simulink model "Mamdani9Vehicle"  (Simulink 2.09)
settings: Solver=ode45  StartTime=0.0  StopTime=50  MaxStep=10  RelTol=1e-3  AbsTol=1e-3
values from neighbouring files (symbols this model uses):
  vd = 45    [VdataM.m]
undefined symbols (not defined in the file or in its folder): sfunyst
libraries: fuzzy x4

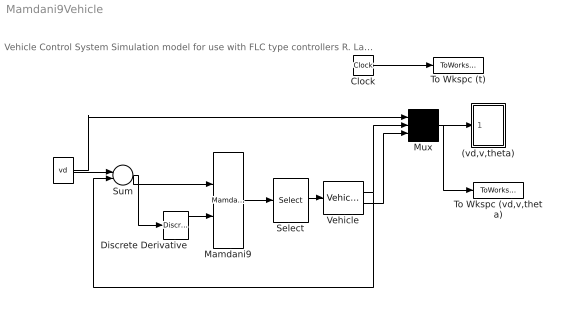
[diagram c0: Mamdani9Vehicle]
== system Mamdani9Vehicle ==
  note: Vehicle Control System Simulation model for use with FLC type controllers R. Langari 3/1/97
  " " : Constant  Value=vd
  (vd,v,theta) : Subsystem  mask(Storage scope.){}
      mask help: Storage scope using MATLAB graph window. Enter plotting ranges and line type.
      mask init:
      | npts = @4; color = @5; ax = [0, @1, @2, @3]; dt=-1;
  Clock : Clock
  Discrete Derivative : fuzzy/Discrete Derivative
  Mamdani9 : fuzzy/Mamdani9
  Mux : Mux  Inputs=3
  Select : fuzzy/Select
  Sum : Sum  Inputs=+-
  To Wkspc (vd,v,theta) : ToWorkspace  VariableName=yout  SampleTime=0
  To Wkspc (t) : ToWorkspace  VariableName=t  SampleTime=0
  Vehicle : fuzzy/Vehicle
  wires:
  Select/1 -> Vehicle/1
  Mux/1 -> (vd,v,theta)/1(x), To Wkspc (vd,v,theta)/1
  Vehicle/1 -> Sum/2, Mux/2
  Vehicle/2 -> Mux/3
  Mamdani9/1 -> Select/1
  " "/1 -> Mux/1, Sum/1
  Discrete Derivative/1 -> Mamdani9/2
  Sum/1 -> Discrete Derivative/1, Mamdani9/1
  Clock/1 -> To Wkspc (t)/1

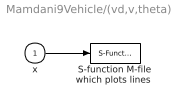
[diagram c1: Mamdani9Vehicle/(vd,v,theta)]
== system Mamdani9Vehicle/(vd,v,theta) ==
  x : Inport  Port=1  PortWidth=-1  SampleTime=-1
  "S-function M-file which plots lines " : S-Function  LoadFcn=sfunyst([],[],[],'LoadBlock')  FunctionName=sfunyst  Parameters=ax, color, npts, dt
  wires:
  x/1 -> "S-function M-file which plots lines "/1
